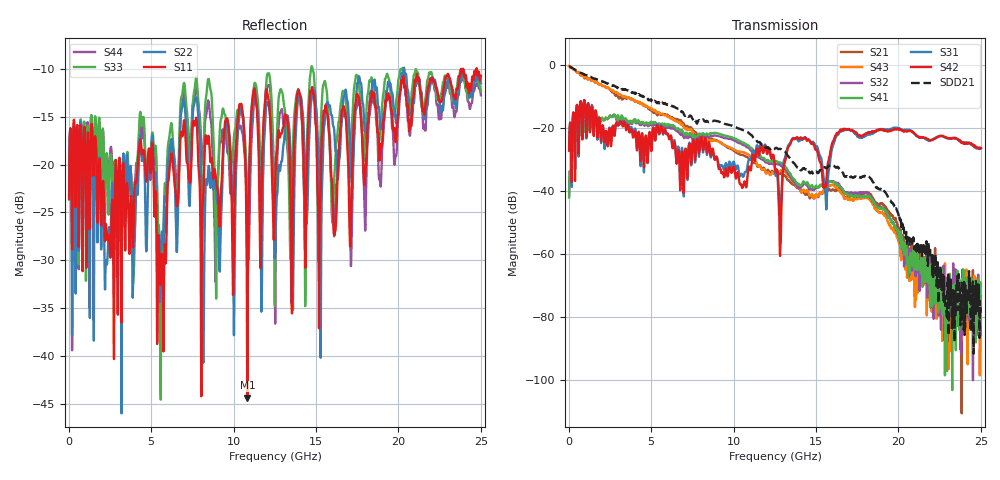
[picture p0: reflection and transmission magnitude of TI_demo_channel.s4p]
! FILE: C:\DATA\DATA\Jose\PCB_104_xcede\N4000_13_SI_12_inches_meas\12_inch_meas\CD4_CD4_Through.s4p
# MHZ S MA R 50.00
! FREQ  S11  S12  S13  S14
!  S21  S22  S23  S24
!  S31  S32  S33  S34
!  S41  S42  S43  S44
!  MAG  ANG  MAG  ANG  MAG  ANG  MAG  ANG
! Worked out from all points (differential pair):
!   1250 points, 20 MHz to 25 GHz, reference 50 ohm
!   strongest paths, dB at 20 MHz, 6.26 GHz, 12.52 GHz, 18.76 GHz, 25 GHz:
!     S42: -27.1, -24.7, -33.1, -20.7, -26.4
!     S31: -27.2, -25.3, -34.1, -20.5, -26.4
!     S41: -42.1, -19.2, -30.6, -45.2, -82.4
!     S32: -41.6, -20.0, -31.3, -44.7, -85.4
!     S43: -0.4, -17.0, -34.2, -46.5, -76.0
!     S21: -0.4, -16.6, -34.1, -44.0, -73.4
!   taken as a pair (ports 3,1 in; 4,2 out), SDD21 dB: -0.4, -13.0, -26.5, -39.2, -77.4
!   lowest |S11| = -44.4 dB at 10.84 GHz (marker M1), VSWR 1.01, Z = 49.6 + j0.44 ohm
!   |S11| at or under -10 dB: start of sweep to 23.8 GHz; 23.92 GHz to 24.72 GHz (800.3 MHz wide, 3.29 % of centre); 24.75 GHz to end of sweep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
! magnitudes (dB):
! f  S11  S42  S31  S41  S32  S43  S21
! 20 MHz  -23.6  -27.1  -27.2  -42.1  -41.6  -0.4  -0.4
! 1.7 GHz  -22.0  -18.7  -18.5  -17.8  -18.2  -5.6  -5.6
! 10.84 GHz  -44.4  -35.3  -32.1  -25.4  -26.2  -28.2  -29.3
! 11.24 GHz  -12.1  -29.5  -27.6  -27.5  -28.3  -30.5  -31.2
! 12.84 GHz  -16.9  -57.2  -43.8  -31.0  -31.9  -33.6  -34.3
! 13.78 GHz  -14.1  -23.2  -23.4  -37.2  -38.0  -38.3  -38.5
! 25 GHz  -10.7  -26.4  -26.4  -82.4  -85.4  -76.0  -73.4
